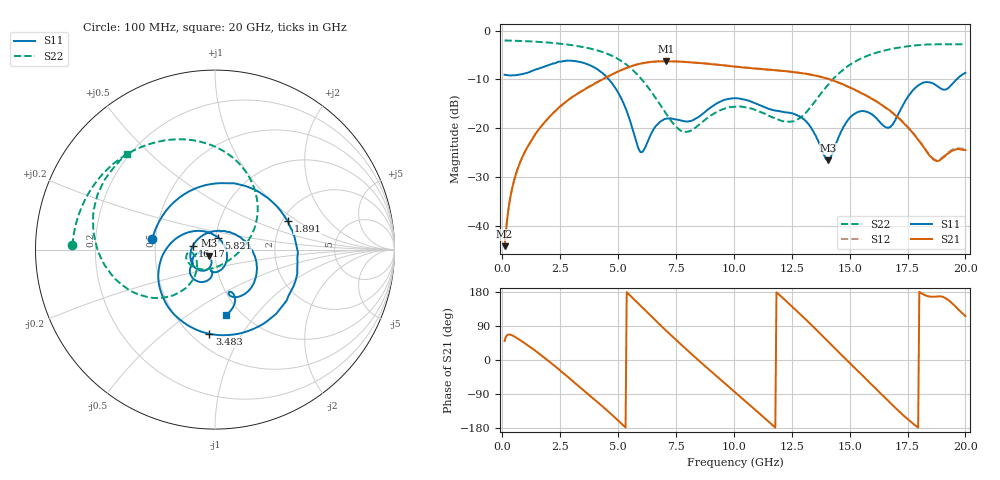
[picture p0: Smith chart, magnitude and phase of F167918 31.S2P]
!  2-Port S-parameters saved by WinCal
! VAR MeasName=S-Parameters (CALIBRATED_DATA) read from VNA (N5242A)
! VAR MeasDate=2016-11-22 10:26:13
! VAR NAME=F167918 31
! VAR FILENAME=F167918 31.S2P
! VAR DATE=2016-11-22 10:26:13
! VAR PHYS_PORTS=1,2
# Hz S DB R 50
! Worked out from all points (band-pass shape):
!   401 points, 100 MHz to 20 GHz, reference 50 ohm
!   highest |S21| = -6.26 dB at 7.065 GHz (marker M1); lowest = -44.2 dB at 100 MHz (marker M2)
!   |S21| within 3 dB of the highest: 4.618 GHz to 13.58 GHz (8.96 GHz wide, 98.5 % of centre)
!   lowest |S11| = -26.6 dB at 14.08 GHz (marker M3), VSWR 1.10, Z = 46.7 - j3.18 ohm
!   |S11| at or under -10 dB: 4.605 GHz to 19.62 GHz (15.01 GHz wide, 124 % of centre)
!   |S22| runs from -20.8 to -2.0 dB; largest |S21 - S12| = 0.003
!   S11 on the Smith chart (normalised r, x): 100 MHz: 0.48, +0.07; 1.891 GHz: 2.15, +0.83; 3.483 GHz: 0.61, -0.73; 5.821 GHz: 1.03, +0.14; 16.17 GHz: 0.78, +0.03; 20 GHz: 0.85, -0.72
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1e8  -9.03 170.3  -44.18 50.1  -44.08 50.1  -2.00 178.3
6.97e8  -9.04 118.7  -27.88 55.5  -27.84 55.2  -2.08 168.5
1.294e9  -8.24 69.5  -22.22 30.5  -22.22 30.3  -2.21 158.8
1.891e9  -7.21 21.1  -18.43 2.6  -18.44 2.5  -2.40 148.7
2.53775e9  -6.34 -28.4  -15.38 -29.9  -15.38 -29.8  -2.68 137.0
3.43325e9  -6.49 -90.6  -12.38 -76.0  -12.32 -75.9  -3.31 119.0
3.483e9  -6.55 -93.9  -12.25 -78.5  -12.18 -78.5  -3.35 117.9
4.478e9  -9.36 -157.8  -9.61 -130.7  -9.56 -130.9  -4.63 93.1
5.82125e9  -23.27 74.4  -6.92 152.0  -6.93 151.8  -8.94 48.8
6.7665e9  -18.89 -69.3  -6.28 95.4  -6.29 95.3  -14.82 12.0
7.065e9  -18.06 -85.3  -6.26 78.1  -6.27 78.1  -16.92 -2.1
8.458e9  -17.74 -96.6  -6.60 0.1  -6.58 0.1  -19.44 -99.6
1.005e10  -13.85 -123.6  -7.34 -85.3  -7.33 -85.2  -15.58 -158.6
1.17415e10  -16.31 -146.8  -8.09 -175.7  -8.06 -175.8  -17.85 -171.7
1.338325e10  -20.29 -168.2  -9.05 90.4  -9.04 90.5  -15.26 -128.7
1.407975e10  -26.56 -133.7  -9.87 48.4  -9.88 48.3  -11.03 -127.9
1.51245e10  -17.32 -119.7  -11.88 -15.2  -11.85 -15.0  -6.64 -145.7
1.616925e10  -17.98 171.2  -14.56 -77.9  -14.56 -77.5  -4.49 -167.1
1.67165e10  -19.78 95.4  -16.27 -110.7  -16.34 -110.1  -3.84 -177.3
1.77115e10  -12.33 -17.1  -20.90 -166.6  -20.77 -165.8  -3.08 165.4
1.87065e10  -11.11 -70.3  -26.62 167.1  -26.48 167.7  -2.79 149.5
2e10  -8.63 -80.8  -24.48 115.7  -24.26 116.0  -2.78 132.6
